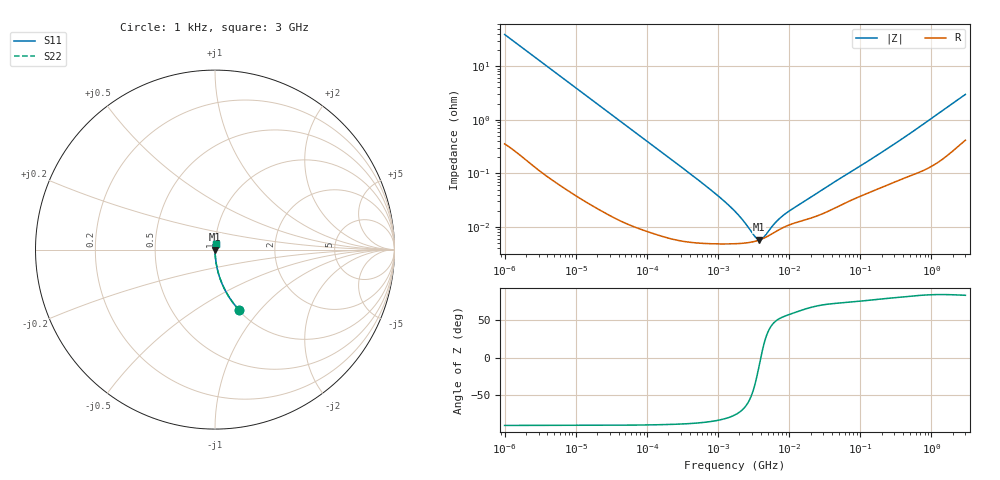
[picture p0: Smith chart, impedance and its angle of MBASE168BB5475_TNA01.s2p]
! MBASE168BB5475_TNA01  S-PARAMETER MODEL  ( Standard Model )
! Model Generated by TAIYO YUDEN Corporation (http://www.ty-top.com)
! Version 1.0
! TAIYO YUDEN Control No. 220601
! Copyright(c) 2014 TAIYO YUDEN CO.,LTD. All Rights Reserved.
! Product Description (link to TY-COMPAS)
! https://ds.yuden.co.jp/TYCOMPAS/or/detail?pn=MBASE168BB5475KTNA01&u=M
! Products Name : Multilayer Ceramic Capacitors
! Characteristics :
!  Capacitance : 4.7 [uF] , Rated Voltage : 16 [V] , TCC : X5R
!  Case Size : 1.6 x 0.8 / 0.063 x 0.031 [mm/inch] , Thickness : 0.8 / 0.031 [mm/inch]
!  (Conditions: Temperature = 25 [degC] , DC Bias Voltage = 0 [V])
! External Node Assignments :
!  1  o---| |---o  2
! GND o---------o GND
! Frequency Range : 1kHz  -  3GHz  [ 401 STEP ]
# MHZ S RI R 50
! Freq[MHz].  S11 Real  S11 Imag  S21 Real  S21 Imag  S12 Real  S12 Imag  S22 Real  S22 Imag
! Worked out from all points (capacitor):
!   401 points, 1 kHz to 3 GHz, reference 50 ohm
!   read as one part in series: C = 4.08 uF near 1.077 kHz
!   lowest |Z| = 5.81 mohm at 3.79 MHz (marker M1)
!   series resonance near 3.997 MHz, so ESL is about 390 pH
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0.001  0.134 -0.3361  0.866 0.3361  0.866 0.3361  0.134 -0.3361
0.001685  0.0529 -0.2193  0.9471 0.2193  0.9471 0.2193  0.0529 -0.2193
0.00306  0.0172 -0.1258  0.9828 0.1258  0.9828 0.1258  0.0172 -0.1258
0.005768  0.00524 -0.0678  0.9948 0.0678  0.9948 0.0678  0.00524 -0.0678
0.01216  0.00138 -0.0324  0.9986 0.0324  0.9986 0.0324  0.00138 -0.0324
0.033275  0.000295 -0.0119  0.9997 0.0119  0.9997 0.0119  0.000295 -0.0119
0.147855  7.71e-05 -0.00271  0.9999 0.00271  0.9999 0.00271  7.71e-05 -0.00271
0.791611  4.9e-05 -0.00049  1 0.00049  1 0.00049  4.9e-05 -0.00049
1.238299  4.85e-05 -0.000295  1 0.000295  1 0.000295  4.85e-05 -0.000295
1.732051  4.88e-05 -0.00019  1 0.00019  1 0.00019  4.88e-05 -0.00019
2.610246  5.09e-05 -8.89e-05  0.9999 8.89e-05  0.9999 8.89e-05  5.09e-05 -8.89e-05
2.812335  5.17e-05 -7.26e-05  0.9999 7.26e-05  0.9999 7.26e-05  5.17e-05 -7.26e-05
3.789741  5.71e-05 -1.06e-05  0.9999 1.06e-05  0.9999 1.06e-05  5.71e-05 -1.06e-05
5.30084  7.03e-05 5.48e-05  0.9999 -5.48e-05  0.9999 -5.48e-05  7.03e-05 5.48e-05
5.711239  7.45e-05 6.86e-05  0.9999 -6.86e-05  0.9999 -6.86e-05  7.45e-05 6.86e-05
7.414467  9.09e-05 0.000115  0.9999 -0.000115  0.9999 -0.000115  9.09e-05 0.000115
8.933959  0.000103 0.000146  0.9999 -0.000146  0.9999 -0.000146  0.000103 0.000146
21.06097  0.00015 0.000343  0.9999 -0.000343  0.9999 -0.000343  0.00015 0.000343
256.0921  0.00064 0.003  0.9994 -0.003  0.9994 -0.003  0.00064 0.003
581.6181  0.00101 0.0063  0.999 -0.0063  0.999 -0.0063  0.00101 0.0063
2489.759  0.00397 0.0247  0.996 -0.0247  0.996 -0.0247  0.00397 0.0247
3000  0.005 0.0292  0.995 -0.0292  0.995 -0.0292  0.005 0.0292
